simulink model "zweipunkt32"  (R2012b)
settings: Solver=ode45  StartTime=0.0  StopTime=50.0  RelTol=1e-3
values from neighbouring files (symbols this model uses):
  denum = denum{:}    [zweipunkt_32.m]
  hy = 0.01    [fuellstnd_3.m]    (also in fuellstnd_31.m; regulator_1.m = 2; zweipunkt_1.m = 20; zweipunkt_2.m = 0)
  Ksensor = 1/1000    (= 0.001)    [zweipunkt_32.m]
  nenner_rueck = nenner_rueck{:}    [fuellstnd_3.m]    (also in fuellstnd_31.m; zweipunkt_31.m; zweipunkt_32.m)
  num = num{:}    [zweipunkt_32.m]
  Ts = 0.001    [fuellstnd_3.m]    (also in fuellstnd_31.m; kalman_d1.m = 0.05; kalman_d2.m = 0.1; kalman_d3.m = 0.1)
  Ustell = 10    [regulator_1.m]    (also in zweipunkt_1.m = 100; zweipunkt_2.m = 100; zweipunkt_21.m = 100; zweipunkt_31.m = 100)
  ysoll = y.signals.values(:,2)    [ohne_kalman_1.m]    (also in zweipunkt_1.m = 500; zweipunkt_2.m = 500; zweipunkt_21.m = 500; zweipunkt_31.m = 500)
  zaehl_rueck = zaehl_rueck{:}    [fuellstnd_3.m]    (also in fuellstnd_31.m; zweipunkt_31.m; zweipunkt_32.m)

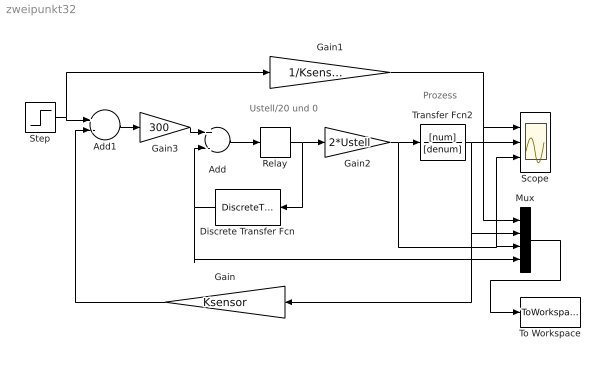
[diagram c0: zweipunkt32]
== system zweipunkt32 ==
  note: Prozess
  note: Ustell/20 und 0
  Add : Sum  Inputs=+-
  Add1 : Sum  Inputs=+-
  Discrete Transfer Fcn : DiscreteTransferFcn  Numerator=[zaehl_rueck]  Denominator=[nenner_rueck]  SampleTime=Ts
  Gain : Gain  Gain=Ksensor  SampleTime=Ts
  Gain1 : Gain  Gain=1/Ksensor
  Gain2 : Gain  Gain=2*Ustell
  Gain3 : Gain  Gain=300
  Mux : Mux
  Relay : Relay  OnSwitchValue=hy  OffSwitchValue=-hy  OnOutputValue=Ustell/20  ZeroCross=off
  Scope : Scope  NumInputPorts=3
  Step : Step  Time=20  After=ysoll  SampleTime=Ts
  To Workspace : ToWorkspace  VariableName=y  SampleTime=-1  SaveFormat=Structure With Time
  Transfer Fcn2 : TransferFcn  Numerator=[num]  Denominator=[denum]
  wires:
  Gain2/1 -> Transfer Fcn2/1, Scope/3, Mux/3
  Transfer Fcn2/1 -> Scope/2, Mux/2, Gain/1
  Step/1 -> Gain1/1, Add1/1
  Add/1 -> Relay/1
  Gain/1 -> Add1/2
  Add1/1 -> Gain3/1
  Mux/1 -> To Workspace/1
  Discrete Transfer Fcn/1 -> Add/2, Mux/4
  Gain1/1 -> Mux/1, Scope/1
  Relay/1 -> Discrete Transfer Fcn/1, Gain2/1
  Gain3/1 -> Add/1
